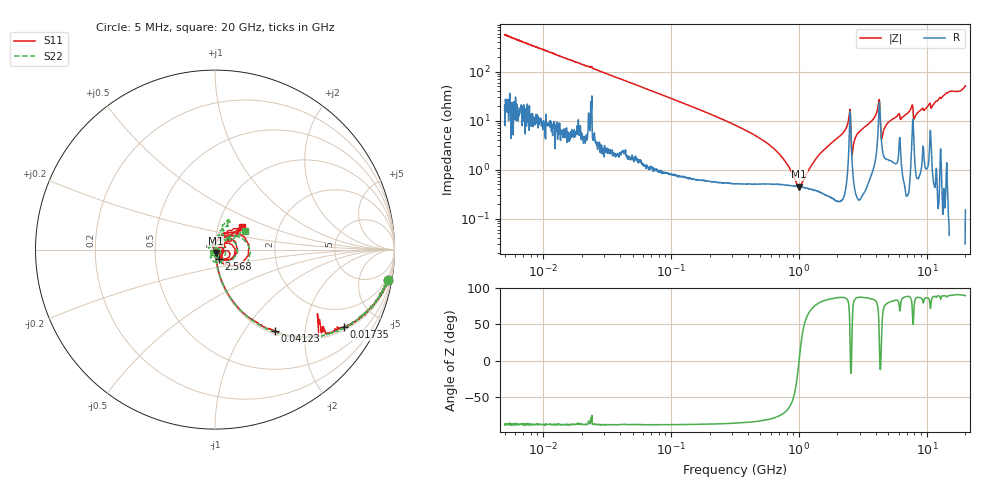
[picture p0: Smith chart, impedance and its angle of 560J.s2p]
!Keysight Technologies,P5008B,MY61100088,A.16.20.02
!Date: Wednesday, November 08, 2023 15:22:28
!Correction: S11(C  2-Port  )
!S21(C  2-Port  )
!S12(C  2-Port  )
!S22(C  2-Port  )
!S2P File: Measurements: S11, S21, S12, S22:Log Frequency Sweep
# Hz S  dB  R 50
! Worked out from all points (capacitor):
!   1601 points, 5 MHz to 20 GHz, reference 50 ohm
!   read as one part in series: C = 56.5 pF near 5.212 MHz
!   lowest |Z| = 451 mohm at 1.005 GHz (marker M1)
!   series resonance near 1.002 GHz, so ESL is about 450 pH
!   S11 on the Smith chart (normalised r, x): 5 MHz: 1, -11; 17.35 MHz: 1.11, -3.26; 41.23 MHz: 1.05, -1.39; 2.568 GHz: 1.04, -0.11; 20 GHz: 1.30, +0.34
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5000000  -0.19 -10.0  -15.24 77.9  -15.24 77.9  -0.19 -9.9
1.734918e7  -1.51 -31.0  -5.77 57.0  -5.76 57.2  -1.50 -31.0
1.995555e7  -1.85 -34.5  -4.94 53.9  -4.93 54.0  -1.83 -34.6
4.123291e7  -5.01 -53.8  -1.86 34.0  -1.82 34.2  -4.98 -54.3
7.964482e7  -9.46 -69.0  -0.60 19.5  -0.60 19.5  -9.47 -69.1
3.162278e8  -21.23 -81.8  -0.08 4.4  -0.08 4.3  -21.39 -82.8
1.004702e9  -33.98 -76.8  -0.05 -1.0  -0.06 -1.0  -36.10 -88.8
1.2621e9  -36.97 -76.7  -0.06 -2.0  -0.06 -2.0  -40.12 -99.8
1.795483e9  -58.27 -173.0  -0.06 -4.0  -0.07 -3.9  -47.87 138.0
2.567557e9  -24.99 -66.9  -0.35 -2.5  -0.36 -2.5  -24.59 -69.7
2.746546e9  -40.30 -139.1  -0.10 -5.5  -0.10 -5.5  -40.27 -102.3
2.938012e9  -39.99 147.3  -0.09 -6.5  -0.09 -6.5  -55.22 150.4
4.201385e9  -16.10 35.9  -1.14 -15.5  -1.14 -15.5  -15.84 23.6
5.037181e9  -38.95 -8.3  -0.13 -10.7  -0.13 -10.7  -33.38 -7.0
5.734159e9  -35.72 19.8  -0.14 -13.1  -0.13 -13.1  -38.53 30.2
7.055393e9  -37.42 -13.1  -0.16 -16.3  -0.15 -16.4  -29.22 159.0
7.948786e9  -24.54 -54.7  -0.34 -15.0  -0.34 -15.1  -25.41 -115.0
8.636175e9  -32.52 -67.2  -0.10 -18.9  -0.10 -19.0  -31.41 -130.4
1.014171e10  -28.99 -34.3  -0.07 -23.6  -0.08 -23.6  -40.50 -153.3
1.442776e10  -15.78 37.4  -0.10 -34.6  -0.10 -34.6  -16.53 66.1
1.812406e10  -21.52 61.1  -0.07 -46.5  -0.07 -46.5  -22.15 50.5
2e10  -14.18 40.7  -0.23 -54.4  -0.24 -54.4  -14.21 31.3
